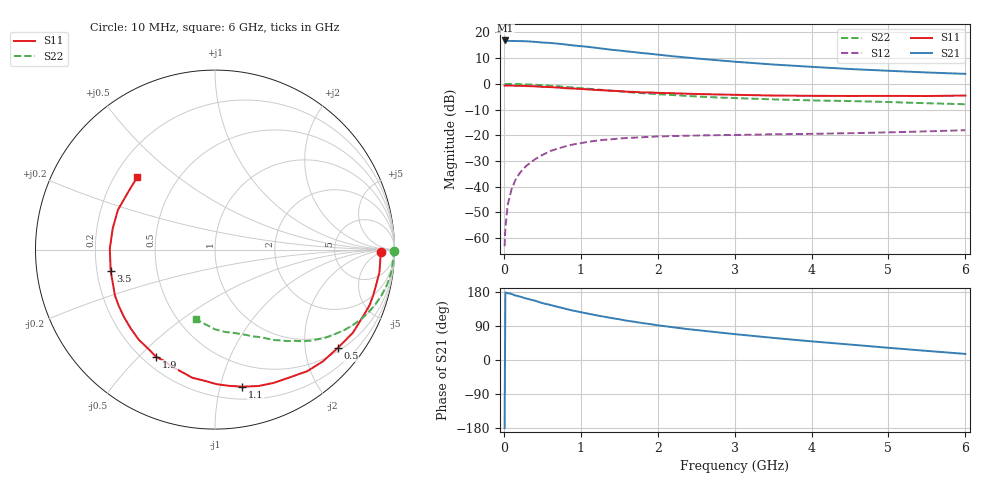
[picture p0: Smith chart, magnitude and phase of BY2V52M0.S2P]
! SIEMENS Small Signal Semiconductors
! BFY420
! Si NPN RF SIEGET Grounded Emitter Transistor in MICRO-X
! VCE = 2.5 V  IC = 2 mA
! Common Emitter S-Parameters:  October  1996
# GHz  S  MA  R  50
!  f  S11  S21  S12  S22
! GHz  MAG  ANG  MAG  ANG  MAG  ANG  MAG  ANG
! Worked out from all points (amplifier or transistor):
!   36 points, 10 MHz to 6 GHz, reference 50 ohm
!   highest |S21| = 16.9 dB at 20 MHz (marker M1)
!   |S21| within 3 dB of that: start of sweep to 1.233 GHz
!   unconditionally stable (mu >= 1): 3.999 GHz to end of sweep
!   at 250 MHz: K = 0.05, MSG = 24.9 dB, |S12| = -33.2 dB
!   at 1.4 GHz: K = 0.29, MSG = 17.4 dB, |S12| = -21.5 dB
!   at 6 GHz: K = 1.24, MAG = 8.0 dB, |S12| = -18.0 dB
!   S11 on the Smith chart (normalised r, x): 10 MHz: 25, -5; 500 MHz: 0.58, -2.74; 1.1 GHz: 0.30, -1.17; 1.9 GHz: 0.25, -0.56; 3.5 GHz: 0.26, -0.09; 6 GHz: 0.29, +0.37
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0.01  0.9258 -0.9  6.97 -179.7  0.0007 101.0  0.9976 -0.4
0.02  0.9225 -1.6  6.981 178.4  0.0016 87.7  0.989 -0.8
0.05  0.9228 -4.2  6.832 176.4  0.0044 93.1  0.9959 -1.9
0.1  0.9247 -7.8  6.833 174.3  0.0089 87.1  0.993 -3.9
0.15  0.9194 -11.8  6.813 170.2  0.0135 81.3  0.9919 -5.9
0.2  0.9177 -15.9  6.776 168.0  0.0179 81.5  0.9885 -7.7
0.3  0.9068 -23.5  6.714 161.8  0.0261 76.7  0.9777 -11.7
0.4  0.897 -31.1  6.568 156.7  0.0339 71.9  0.9615 -15.5
0.5  0.8764 -38.7  6.365 150.2  0.0414 68.2  0.9433 -19.0
0.6  0.8656 -46.0  6.249 145.4  0.0492 64.2  0.9226 -22.4
0.8  0.8246 -59.7  5.835 135.1  0.0612 56.3  0.8745 -28.8
0.9  0.8115 -66.2  5.597 130.3  0.0663 53.0  0.8508 -31.6
1.1  0.7788 -78.7  5.235 122.1  0.0748 47.0  0.803 -36.8
1.4  0.7321 -95.0  4.598 110.7  0.0837 39.7  0.7381 -43.4
1.6  0.7047 -105.7  4.279 103.7  0.0887 35.4  0.695 -47.2
1.9  0.6822 -118.7  3.846 94.8  0.0936 30.3  0.6459 -52.1
2.2  0.6575 -130.3  3.439 86.4  0.0968 26.2  0.6067 -56.3
2.8  0.6215 -149.5  2.859 72.6  0.1009 20.8  0.5425 -63.7
3.5  0.5934 -168.5  2.38 58.4  0.1047 17.1  0.4997 -71.2
4.5  0.5819 168.2  1.944 40.8  0.11 14.3  0.4629 -82.8
5.5  0.5805 146.5  1.665 24.0  0.1195 13.0  0.4201 -97.1
6  0.5927 136.8  1.566 16.1  0.1256 11.9  0.4022 -105.5
